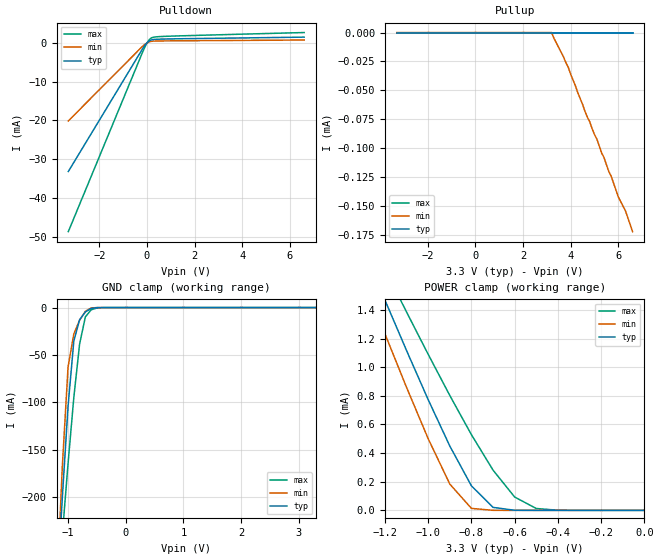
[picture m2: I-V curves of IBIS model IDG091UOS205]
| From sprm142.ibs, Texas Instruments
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[Model]   IDG091UOS205
| Open drain output with input buffer
Model_type   I/O_open_drain
Enable   Active-Low
Polarity   Non-Inverting
| signals   A, GZ, Y
Vmeas = 1.5
Vinh = 2.0
Vinl = 0.80
|   typ   min   max
C_comp   3.010p   2.992p   3.013p
|   typ   min   max
[Temperature Range]   25   -40   125
|   typ   min   max
[Voltage Range]   3.30V   3.00V   3.60V
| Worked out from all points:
|   slope of the pulldown table from 0 to 0.495 V, typ, clamps not added: 511 ohm
|   GND clamp passes 1 mA (typ) near -0.60 V on its own axis
|   POWER clamp passes 1 mA (typ) near -1.07 V on its own axis
[Pulldown]
|   Voltage   I(typ)   I(min)   I(max)
-3.3V     -33.16mA   -20.11mA   -48.66mA
-200mV    -1.676mA   -953uA     -2.637mA
0V        0A         0A         -1uA
100mV     530uA      281uA      888uA
300mV     907uA      480uA      1.509mA
700mV     1.004mA    523uA      1.686mA
6.6V      1.5mA      758uA      2.684mA
[GND_clamp]
|   Voltage   I(typ)   I(min)   I(max)
-3.3V     -2.799A    -3.633A    -2.114A
-1.2V     -308mA     -306.3mA   -319.5mA
-1.1V     -201.1mA   -168.5mA   -240.5mA
-1V       -104.1mA   -62.73mA   -164.6mA
-900mV    -35.35mA   -27.81mA   -94.84mA
-800mV    -12.85mA   -13.43mA   -38.62mA
-700mV    -4.694mA   -3.964mA   -9.888mA
-600mV    -918uA     -456.8uA   -2.377mA
-500mV    -84.38uA   -21.55uA   -425.6uA
-400mV    -4.731uA   -483.2nA   -51.5uA
3.3V      266.4pA    177.6pA    62.26nA
[Pullup]
|   Voltage   I(typ)   I(min)   I(max)
-3.3V     0A         0A         0A
3.2V      0A         0A         0A
3.9V      0A         -30uA      0A
4.6V      0A         -68uA      0A
4.8V      0A         -77uA      0A
5.1V      0A         -92uA      0A
5.3V      0A         -104uA     0A
5.4V      0A         -108uA     0A
5.7V      0A         -124uA     0A
6V        0A         -142uA     0A
6.3V      0A         -154uA     0A
6.6V      0A         -172uA     0A
[POWER_clamp]
|   Voltage   I(typ)   I(min)   I(max)
-3.3V     9.284mA    9.572mA    8.301mA
-1.3V     1.827mA    1.615mA    1.99mA
-1.2V     1.468mA    1.233mA    1.686mA
-1.1V     1.116mA    858.6uA    1.385mA
-1V       773.2uA    500.3uA    1.09mA
-900mV    449.2uA    183.5uA    802.4uA
-800mV    171.1uA    13.68uA    528.5uA
-700mV    20.77uA    148.8nA    280.9uA
-600mV    664.9nA    1.688nA    93uA
-500mV    16.92nA    266.4pA    13.02uA
-400mV    710.5pA    266.4pA    939.2nA
0V        310.9pA    177.6pA    3.153nA
[Ramp]
|   I(typ)   I(min)   I(max)
dV/dt_r   0.028/4.234n   0.027/6.763n   0.030/2.474n
dV/dt_f   1.970/4.234n   1.782/6.763n   2.154/2.474n
R_load = 25000ohms
